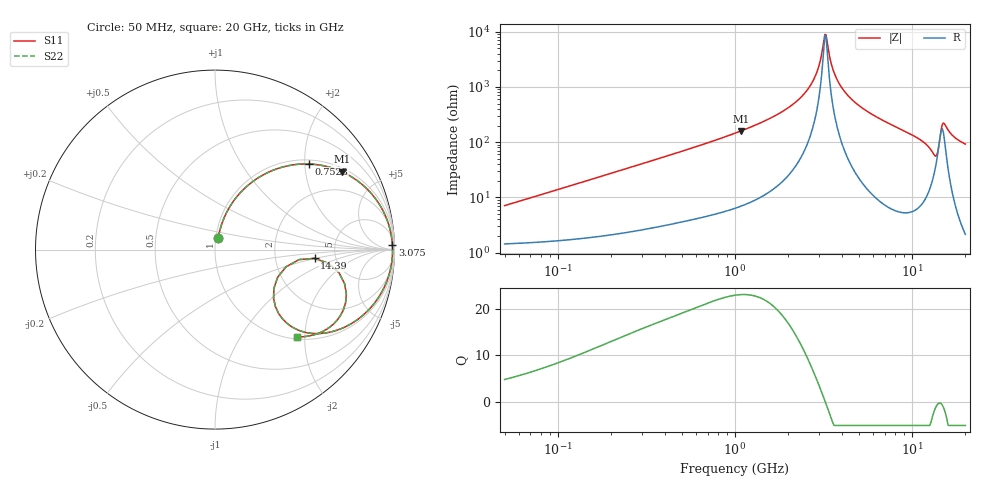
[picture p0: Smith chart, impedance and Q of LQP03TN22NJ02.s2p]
!Murata Part Number: LQP03TN22NJ02
!These Parameters are Measured in Series Mode Connection
!  o--[Z]--o
!Port1  Port2
!  o-------o
!Freq. Start=50[MHz] Stop=20[GHz], 401[Steps]
# Hz S RI R 50
!Freq.(Hz) S11(Real) S11(Imag) S21(Real) S21(Imag) S12(Real) S12(Imag) S22(Real) S22(Imag)
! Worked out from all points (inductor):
!   401 points, 50 MHz to 20 GHz, reference 50 ohm
!   read as one part in series: L = 22 nH near 51.52 MHz
!   highest Q = 23 at 1.078 GHz (marker M1), where L = 23.4 nH
!   self-resonance near 3.217 GHz
!   S11 on the Smith chart (normalised r, x): 50 MHz: 1.03, +0.14; 752.3 MHz: 1.10, +2.09; 3.075 GHz: 31, +68; 14.39 GHz: 3.44, -0.49; 20 GHz: 1.04, -1.84
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5e7  0.0187 0.0672  0.9813 -0.0672  0.9813 -0.0672  0.0187 0.0672
1.364002e8  0.0496 0.1742  0.9504 -0.1742  0.9504 -0.1742  0.0496 0.1742
3.721004e8  0.2167 0.3839  0.7833 -0.3839  0.7833 -0.3839  0.2167 0.3839
7.523192e8  0.5226 0.4769  0.4774 -0.4769  0.4774 -0.4769  0.5226 0.4769
1e9  0.6708 0.4486  0.3292 -0.4486  0.3292 -0.4486  0.6708 0.4486
1.077769e9  0.708 0.4335  0.292 -0.4335  0.292 -0.4335  0.708 0.4335
1.962148e9  0.9304 0.2272  0.0696 -0.2272  0.0696 -0.2272  0.9304 0.2272
2.728004e9  0.9822 0.0797  0.0178 -0.0797  0.0178 -0.0797  0.9822 0.0797
2.940159e9  0.987 0.0451  0.013 -0.0451  0.013 -0.0451  0.987 0.0451
3.075291e9  0.9886 0.0242  0.0114 -0.0242  0.0114 -0.0242  0.9886 0.0242
3.168813e9  0.9892 0.0102  0.0108 -0.0102  0.0108 -0.0102  0.9892 0.0102
3.265178e9  0.9894 -0.00378  0.0106 0.00378  0.0106 0.00378  0.9894 -0.00378
3.626126e9  0.9869 -0.0528  0.0131 0.0528  0.0131 0.0528  0.9869 -0.0528
4.149438e9  0.9761 -0.116  0.0239 0.116  0.0239 0.116  0.9761 -0.116
5.273168e9  0.9345 -0.2268  0.0655 0.2268  0.0655 0.2268  0.9345 -0.2268
7.442007e9  0.8159 -0.3729  0.1841 0.3729  0.1841 0.3729  0.8159 -0.3729
1.183995e10  0.4766 -0.4533  0.5234 0.4533  0.5234 0.4533  0.4766 -0.4533
1.334722e10  0.3264 -0.2718  0.6736 0.2718  0.6736 0.2718  0.3264 -0.2718
1.438523e10  0.5547 -0.0488  0.4453 0.0488  0.4453 0.0488  0.5547 -0.0488
1.550395e10  0.7275 -0.2964  0.2725 0.2964  0.2725 0.2964  0.7275 -0.2964
1.696185e10  0.6213 -0.4442  0.3787 0.4442  0.3787 0.4442  0.6213 -0.4442
2e10  0.4593 -0.4869  0.5407 0.4869  0.5407 0.4869  0.4593 -0.4869
